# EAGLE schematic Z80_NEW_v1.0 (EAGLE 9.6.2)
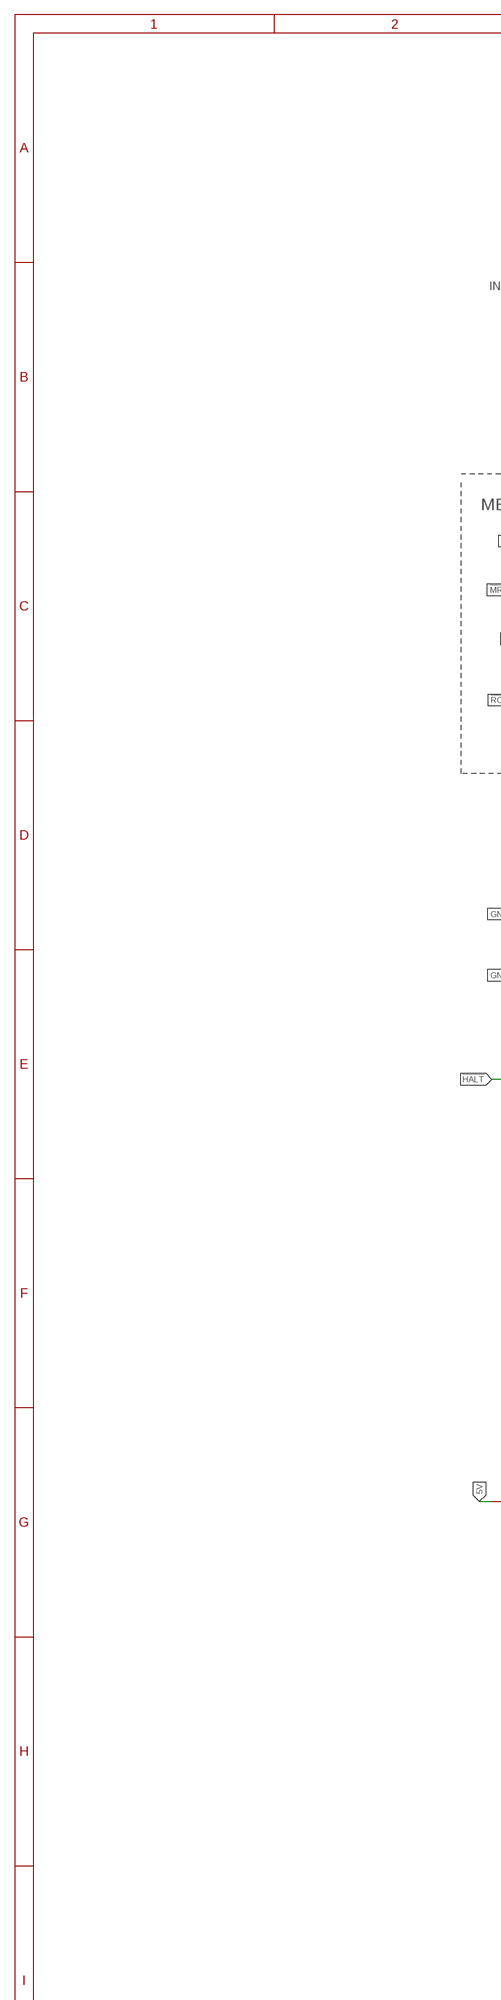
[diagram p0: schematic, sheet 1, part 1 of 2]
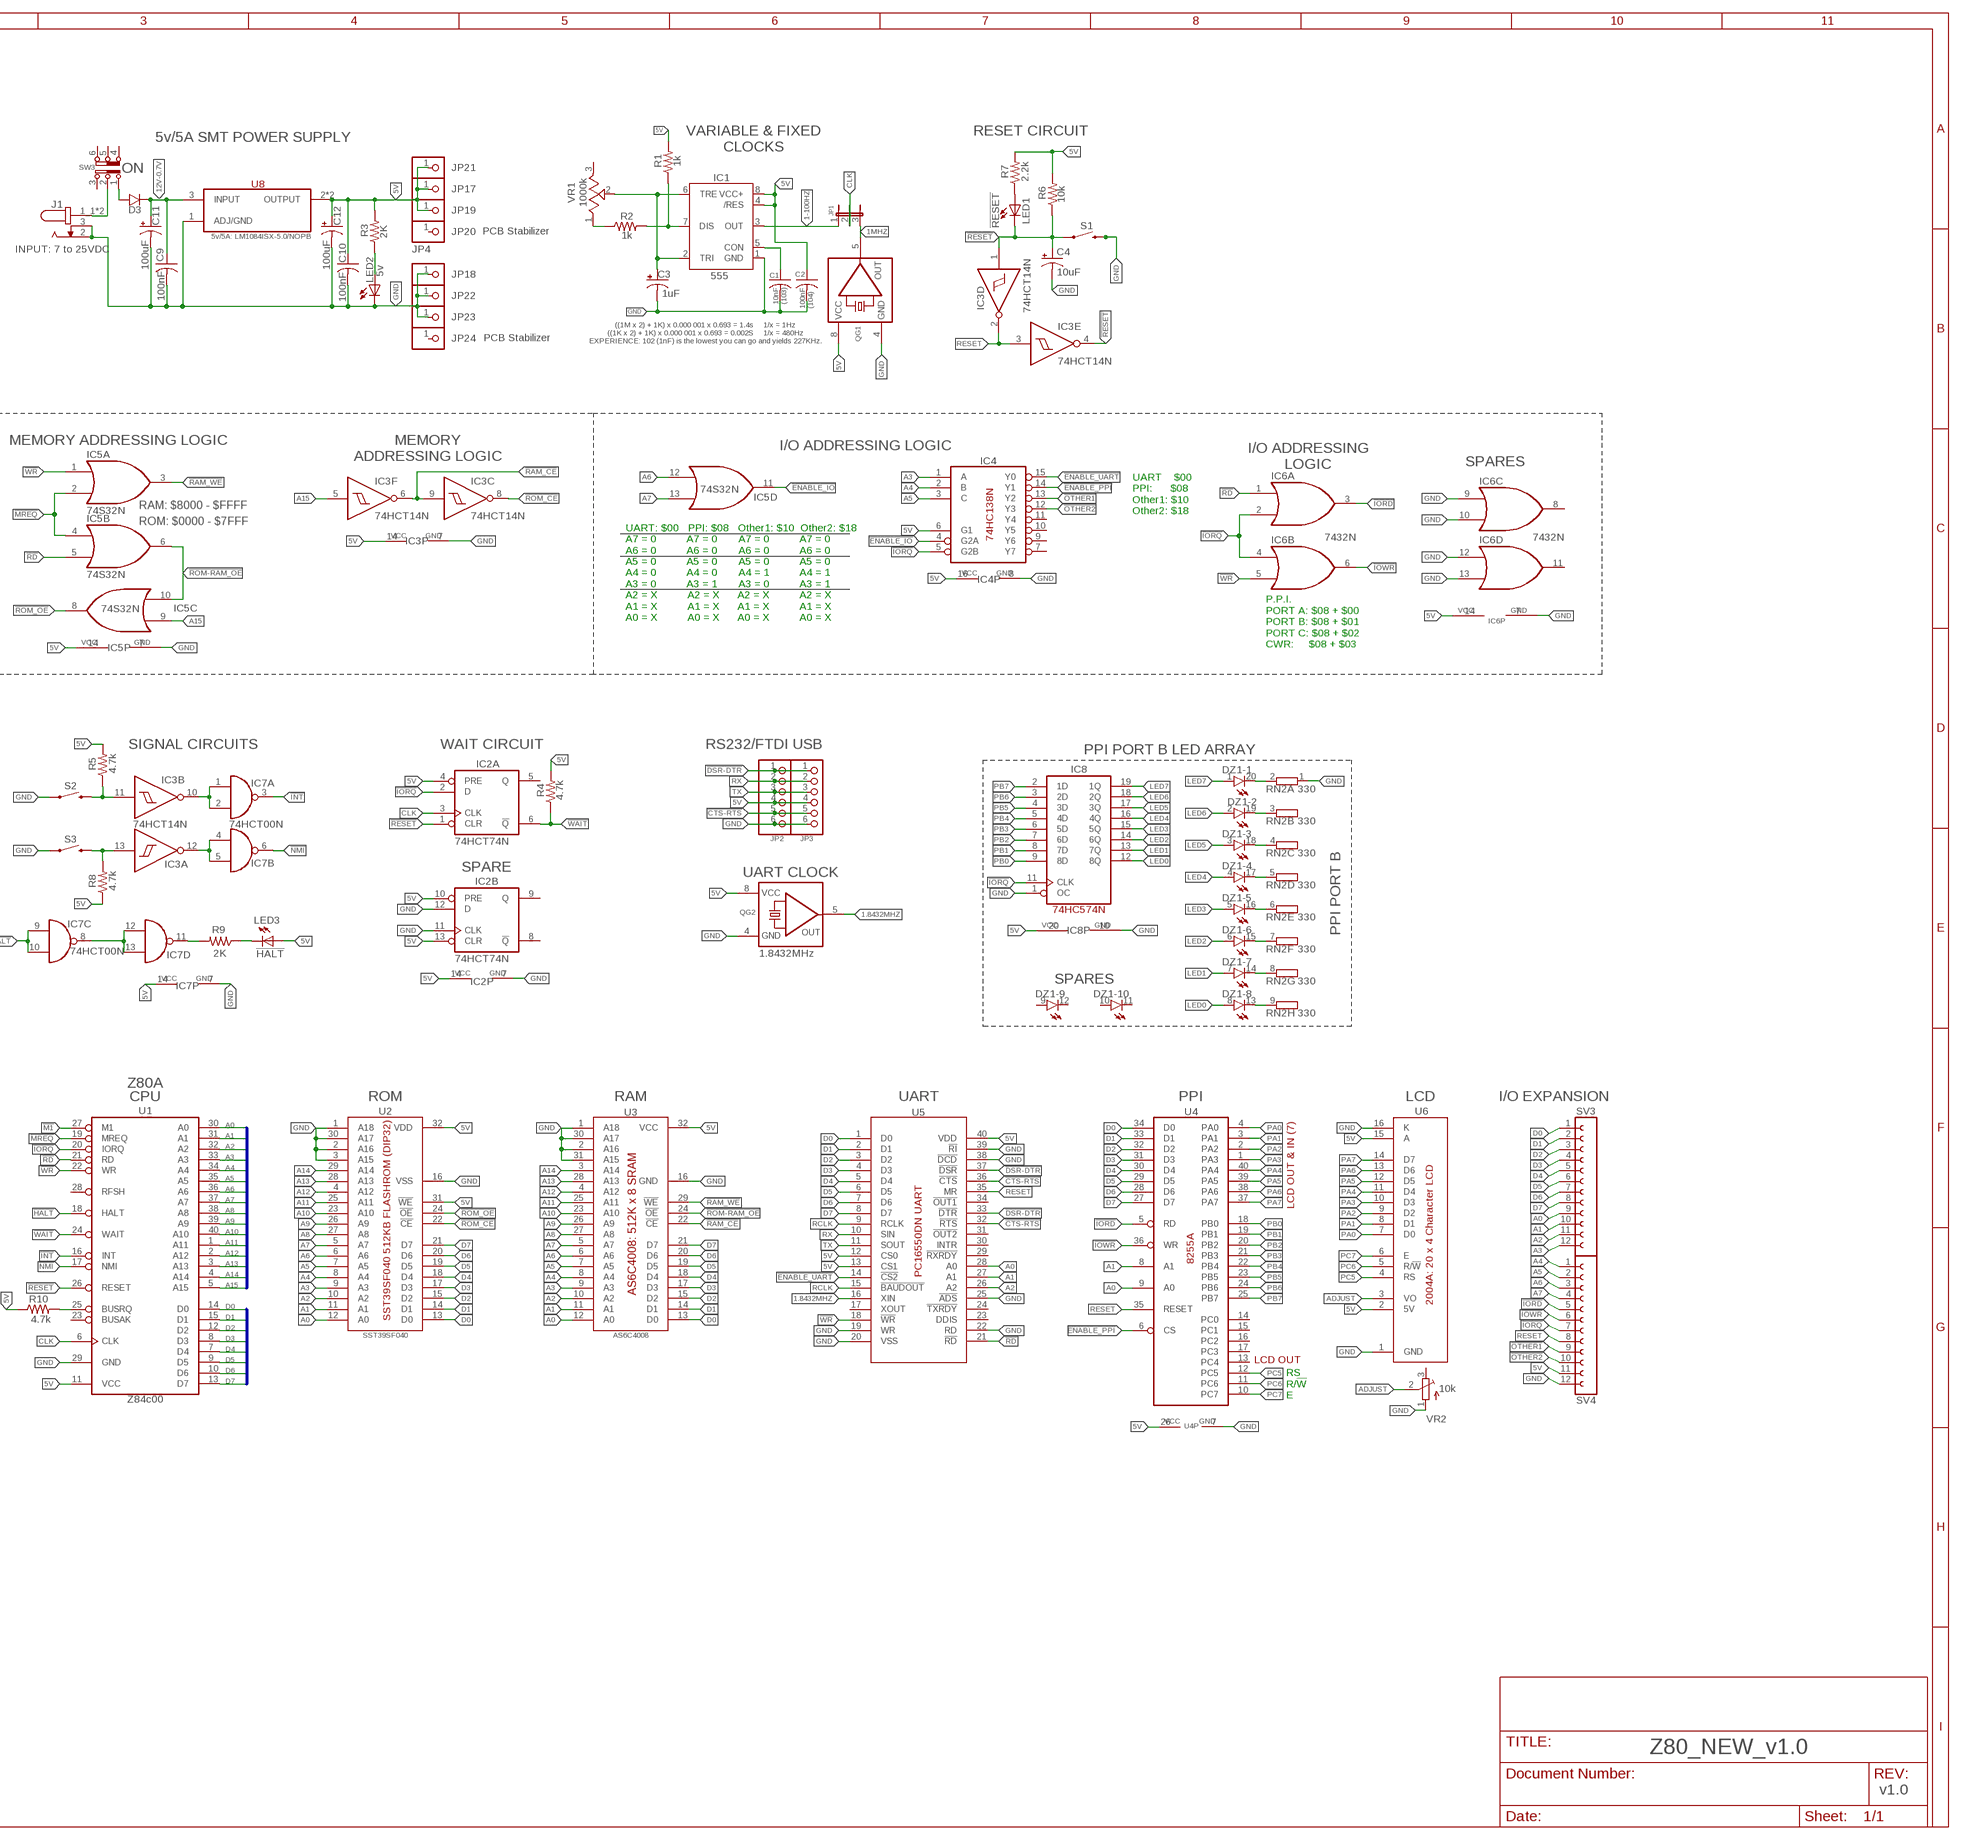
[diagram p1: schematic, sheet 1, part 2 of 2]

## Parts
C1  0.01uF  C-USC1206  [C1206]
C2  0.01uF  C-USC1206  [C1206]
C3  1uF  CPOL-USE2-5  [E2-5]
C4  10uF  CPOL-USE2-5  [E2-5]
C9  100nF  C-USC1206  [C1206]
C10  100nF  C-USC1206  [C1206]
C11  100uF  CPOL-USF  [PANASONIC_F]
C12  100uF  CPOL-USF  [PANASONIC_F]
D3  D1  DIODE_5V5A  [DIODE_5V5A]
DZ1  LB10  [LB10]
IC1  555  555P  [DIP08]
IC2  74HCT74N  [DIL14]
IC3  74HCT14N  [DIL14]
IC4  74HC138N  [DIL16]
IC5  74S32N  [DIL14]
IC6  7432N  [DIL14]
IC7  74HCT00N  [DIL14]
IC8  74HC574N  [DIL20]
J1  PRT-12748  [SPARKFUN_PRT-12748]
JP1  JP2E  [JP2]
JP2  PINHD-1X6  [1X06]
JP3  PINHD-1X6  [1X06]
JP17  PINHD-1X1  [1X01]
JP18  PINHD-1X1  [1X01]
JP19  PINHD-1X1  [1X01]
JP20  JP4  PINHD-1X1  [1X01]
JP21  PINHD-1X1  [1X01]
JP22  PINHD-1X1  [1X01]
JP23  PINHD-1X1  [1X01]
JP24  PINHD-1X1  [1X01]
LED1  !RESET!  LED3MM  [LED3MM]
LED2  5v  LEDCHIPLED_1206  [CHIPLED_1206]
LED3  !HALT!  LEDCHIPLED_1206  [CHIPLED_1206]
QG1  QG5460  [DIL08S]
QG2  1.8432MHz  QG5460  [DIL08S]
R1  1k  R-US_R1206  [R1206]
R2  1k  R-US_R1206  [R1206]
R3  2K  R-US_R1206  [R1206]
R4  4.7k  R-US_R1206  [R1206]
R5  4.7k  R-US_R1206  [R1206]
R6  10k  R-US_R1206  [R1206]
R7  2.2k  R-US_R1206  [R1206]
R8  4.7k  R-US_R1206  [R1206]
R9  2K  R-US_R1206  [R1206]
R10  4.7k  R-US_R1206  [R1206]
RN2  330  GE08R  [SIL9]
S1  MOMENTARY_SWITCH"  [MOMENTARY_SWITCH]
S2  MOMENTARY_SWITCH"  [MOMENTARY_SWITCH]
S3  MOMENTARY_SWITCH"  [MOMENTARY_SWITCH]
SV3  FE12W  [FE12W]
SV4  FE12W  [FE12W]
SW3  JS202011SCQN  [JS202011SCQN]
U1  Z80CPU  [DIL40]
U2  SST39SF040_DIP32  [DIL32]
U3  ALLIANCE_AS6C4008  [DIL32]
U4  8255A  [DIL40]
U5  PC16550DN/NOPB  [N40A]
U6  20X4LCD_2004A  [20X4LCD_2004A]
U8  LM1084ISX-5.0/NOPB  [TO254P1524X483-4N]
VR1  1000k  3352T-1-105LF  [TRIM_3352T-1-105LF]
VR2  10k  TRIMPOT3386  [TRIM-3386]

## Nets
1-100HZ: IC1.3(OUT) JP1.1
1.8432MHZ: QG2.5(OUT) U5.16(XIN)
1MHZ: JP1.3 QG1.5(OUT)
5V [Power]: C2.1 C10.1 C12.+ IC1.4(/RES) IC1.8(VCC+) IC2.4(A:PRE) IC2.10(B:PRE) IC2.13(B:CLR) IC2.14(P:VCC) IC3.14(P:VCC) IC4.6(G1) IC4.16(VCC) IC5.14(P:VCC) IC6.14(P:VCC) IC7.14(P:VCC) IC8.20(VCC) JP2.4 JP3.4 JP17.1 JP19.1 JP21.1 LED3.A QG1.8(VCC) QG2.8(VCC) R1.2 R3.2 R4.2 R5.2 R6.2 R7.2 R8.1 R10.1 SV4.11 U1.11(VCC) U2.31(!WE!) U2.32(VDD) U3.32(VCC) U4.26(VCC) U5.12(CS0) U5.13(CS1) U5.40(VDD) U6.2(5V) U6.15(A) U8.2(OUTPUT) U8.4(OUTPUT)
12V-0.7V: C9.1 C11.+ D3.C U8.3(INPUT)
!BUSRQ!: R10.2 U1.25(BUSRQ)
!CTS-RTS!: JP2.5 JP3.5 U5.32(!RTS) U5.36(!CTS)
!DSR-DTR!: JP2.1 JP3.1 U5.33(!DTR) U5.37(!DSR)
!ENABLE_IO!: IC4.4(G2A) IC5.11(D:O)
!ENABLE_PPI!: IC4.14(Y1) U4.6(CS)
!ENABLE_UART!: IC4.15(Y0) U5.14(!CS2)
!HALT!: IC7.9(C:I0) IC7.10(C:I1) U1.18(HALT)
!INT!: IC7.3(A:O) U1.16(INT)
!IORD!: IC6.3(A:O) SV4.5 U4.5(RD)
!IORQ!: IC2.2(A:D) IC4.5(G2B) IC6.2(A:I1) IC6.4(B:I0) IC8.11(CLK) SV4.7 U1.20(IORQ)
!IOWR!: IC6.6(B:O) SV4.6 U4.36(WR)
!M1!: U1.27(M1)
!MREQ!: IC5.2(A:I1) IC5.4(B:I0) U1.19(MREQ)
!NMI!: IC7.6(B:O) U1.17(NMI)
!OTHER1!: IC4.13(Y2) SV4.9
!OTHER2!: IC4.12(Y3) SV4.10
!RAM_CE!: IC3.6(F:O) IC3.9(C:I) U3.22(!CE!)
!RAM_WE!: IC5.3(A:O) U3.29(!WE!)
!RD!: IC5.5(B:I1) IC6.1(A:I0) U1.21(RD) U5.21(!RD)
!RESET!: C4.+ IC2.1(A:CLR) IC3.1(D:I) IC3.4(E:O) LED1.K(C) R6.1 S1.1 U1.26(RESET)
!ROM-RAM_OE!: IC5.6(B:O) IC5.10(C:I1) U3.24(!OE!)
!ROM_CE!: IC3.8(C:O) U2.22(!CE!)
!ROM_OE!: IC5.8(C:O) U2.24(!OE!)
!WAIT!: IC2.6(A:!Q) R4.1 U1.24(WAIT)
!WR!: IC5.1(A:I0) IC6.5(B:I1) U1.22(WR) U5.18(!WR)
A0: SV3.9 U1.30(A0) U2.12(A0) U3.12(A0) U4.9(A0) U5.28(A0)
A1: SV3.10 U1.31(A1) U2.11(A1) U3.11(A1) U4.8(A1) U5.27(A1)
A2: SV3.11 U1.32(A2) U2.10(A2) U3.10(A2) U5.26(A2)
A3: IC4.1(A) SV3.12 U1.33(A3) U2.9(A3) U3.9(A3)
A4: IC4.2(B) SV4.1 U1.34(A4) U2.8(A4) U3.8(A4)
A5: IC4.3(C) SV4.2 U1.35(A5) U2.7(A5) U3.7(A5)
A6: IC5.12(D:I0) SV4.3 U1.36(A6) U2.6(A6) U3.6(A6)
A7: IC5.13(D:I1) SV4.4 U1.37(A7) U2.5(A7) U3.5(A7)
A8: U1.38(A8) U2.27(A8) U3.27(A8)
A9: U1.39(A9) U2.26(A9) U3.26(A9)
A10: U1.40(A10) U2.23(A10) U3.23(A10)
A11: U1.1(A11) U2.25(A11) U3.25(A11)
A12: U1.2(A12) U2.4(A12) U3.4(A12)
A13: U1.3(A13) U2.28(A13) U3.28(A13)
A14: U1.4(A14) U2.29(A14) U3.3(A14)
A15: IC3.5(F:I) IC5.9(C:I0) U1.5(A15)
ADJUST: U6.3(VO) VR2.2(S)
CLK: IC2.3(A:CLK) JP1.2 U1.6(CLK)
D0: SV3.1 U1.14(D0) U2.13(D0) U3.13(D0) U4.34(D0) U5.1(D0)
D1: SV3.2 U1.15(D1) U2.14(D1) U3.14(D1) U4.33(D1) U5.2(D1)
D2: SV3.3 U1.12(D2) U2.15(D2) U3.15(D2) U4.32(D2) U5.3(D2)
D3: SV3.4 U1.8(D3) U2.17(D3) U3.17(D3) U4.31(D3) U5.4(D3)
D4: SV3.5 U1.7(D4) U2.18(D4) U3.18(D4) U4.30(D4) U5.5(D4)
D5: SV3.6 U1.9(D5) U2.19(D5) U3.19(D5) U4.29(D5) U5.6(D5)
D6: SV3.7 U1.10(D6) U2.20(D6) U3.20(D6) U4.28(D6) U5.7(D6)
D7: SV3.8 U1.13(D7) U2.21(D7) U3.21(D7) U4.27(D7) U5.8(D7)
GND [Power]: C1.2 C2.2 C3.- C4.- C9.2 C10.2 C11.- C12.- IC1.1(GND) IC2.7(P:GND) IC2.11(B:CLK) IC2.12(B:D) IC3.7(P:GND) IC4.8(GND) IC5.7(P:GND) IC6.7(P:GND) IC6.9(C:I0) IC6.10(C:I1) IC6.12(D:I0) IC6.13(D:I1) IC7.7(P:GND) IC8.1(OC) IC8.10(GND) J1.2 J1.3 JP2.6 JP3.6 JP18.1 JP22.1 JP23.1 LED2.C QG1.4(GND) QG2.4(GND) RN2.1 S1.3 S2.1 S3.1 SV4.12 U1.29(GND) U2.1(A18) U2.2(A16) U2.3(A15) U2.16(VSS) U2.30(A17) U3.1(A18) U3.2(A16) U3.16(GND) U3.30(A17) U3.31(A15) U4.7(GND) U5.19(WR) U5.20(VSS) U5.22(RD) U5.25(!ADS) U5.38(!DCD) U5.39(!RI) U6.1(GND) U6.16(K) U8.1(ADJ/GND) VR2.1(A)
LED0: DZ1.8(-8:A) IC8.12(8Q)
LED1: DZ1.7(-7:A) IC8.13(7Q)
LED2: DZ1.6(-6:A) IC8.14(6Q)
LED3: DZ1.5(-5:A) IC8.15(5Q)
LED4: DZ1.4(-4:A) IC8.16(4Q)
LED5: DZ1.3(-3:A) IC8.17(3Q)
LED6: DZ1.2(-2:A) IC8.18(2Q)
LED7: DZ1.1(-1:A) IC8.19(1Q)
N$1: LED1.A R7.1
N$2: IC1.7(DIS) R1.1 R2.2
N$3: C3.+ IC1.2(TRI) IC1.6(TRE) VR1.2(WIPER)
N$4: C1.1 IC1.5(CON)
N$5: D3.A SW3.1
N$6: R2.1 VR1.1(CCW)
N$8: J1.1_1 J1.1_2 SW3.2
N$9: LED2.A R3.1
N$10: IC3.10(B:O) IC7.1(A:I0) IC7.2(A:I1)
N$11: DZ1.20(-1:C) RN2.2
N$12: IC3.12(A:O) IC7.4(B:I0) IC7.5(B:I1)
N$13: DZ1.19(-2:C) RN2.3
N$14: IC7.8(C:O) IC7.12(D:I0) IC7.13(D:I1)
N$15: DZ1.18(-3:C) RN2.4
N$16: LED3.C R9.1
N$17: IC7.11(D:O) R9.2
N$18: DZ1.17(-4:C) RN2.5
N$19: IC3.11(B:I) R5.1 S2.3
N$20: IC3.13(A:I) R8.2 S3.3
N$22: DZ1.16(-5:C) RN2.6
N$23: DZ1.15(-6:C) RN2.7
N$24: DZ1.14(-7:C) RN2.8
N$25: DZ1.13(-8:C) RN2.9
PA0: U4.4(PA0) U6.7(D0)
PA1: U4.3(PA1) U6.8(D1)
PA2: U4.2(PA2) U6.9(D2)
PA3: U4.1(PA3) U6.10(D3)
PA4: U4.40(PA4) U6.11(D4)
PA5: U4.39(PA5) U6.12(D5)
PA6: U4.38(PA6) U6.13(D6)
PA7: U4.37(PA7) U6.14(D7)
PB0: IC8.9(8D) U4.18(PB0)
PB1: IC8.8(7D) U4.19(PB1)
PB2: IC8.7(6D) U4.20(PB2)
PB3: IC8.6(5D) U4.21(PB3)
PB4: IC8.5(4D) U4.22(PB4)
PB5: IC8.4(3D) U4.23(PB5)
PB6: IC8.3(2D) U4.24(PB6)
PB7: IC8.2(1D) U4.25(PB7)
PC5: U4.12(PC5) U6.4(RS)
PC6: U4.11(PC6) U6.5(R/!W!)
PC7: U4.10(PC7) U6.6(E)
RCLK: U5.9(RCLK) U5.15(!BAUDOUT)
RESET: IC3.2(D:O) IC3.3(E:I) SV4.8 U4.35(RESET) U5.35(MR)
RX: JP2.2 JP3.2 U5.10(SIN)
TX: JP2.3 JP3.3 U5.11(SOUT)
Unconnected: DZ1.9(-9:A) DZ1.10(-10:A) DZ1.11(-10:C) DZ1.12(-9:C) IC2.5(A:Q) IC2.8(B:!Q) IC2.9(B:Q) IC4.7(Y7) IC4.9(Y6) IC4.10(Y5) IC4.11(Y4) IC6.8(C:O) IC6.11(D:O) JP20.1 JP24.1 SW3.3 SW3.4 SW3.5 SW3.6 U1.23(BUSAK) U1.28(RFSH) U4.13(PC4) U4.14(PC0) U4.15(PC1) U4.16(PC2) U4.17(PC3) U5.17(XOUT) U5.23(DDIS) U5.24(!TXRDY) U5.29(!RXRDY) U5.30(INTR) U5.31(!OUT2) U5.34(!OUT1) VR1.3(CW) VR2.3(E)

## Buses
ADDRESSBUS:A0,A1,A2,A3,A4,A5,A6,A7,A8,A9,A10,A11,A12,A13,A14,A15
DATABUS:D0,D1,D2,D3,D4,D5,D6,D7

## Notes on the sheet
- RESET CIRCUIT
- 5v/5A SMT POWER SUPPLY
- VARIABLE & FIXED
  CLOCKS
- ON
- PCB Stabilizer
- 5v/5A: LM1084ISX-5.0/NOPB
- INPUT: 7 to 25VDC
- 10nF
  (103)
- 100nF
  (104)
- PCB Stabilizer
- ((1M x 2) + 1K) x 0.000 001 x 0.693 = 1.4s     1/x = 1Hz
  ((1K x 2) + 1K) x 0.000 001 x 0.693 = 0.002S     1/x = 480Hz
  EXPERIENCE: 102 (1nF) is the lowest you can go and yields 227KHz.
- MEMORY ADDRESSING LOGIC
- I/O ADDRESSING LOGIC
- I/O ADDRESSING
  LOGIC
- MEMORY
  ADDRESSING LOGIC
- SPARES
- RAM: $8000 - $FFFF
- UART    $00   
  PPI:      $08  
  Other1: $10  
  Other2: $18
- ROM: $0000 - $7FFF
- UART: $00   PPI: $08   Other1: $10  Other2: $18
  A7 = 0          A7 = 0       A7 = 0          A7 = 0 
  A6 = 0          A6 = 0       A6 = 0          A6 = 0
  A5 = 0          A5 = 0       A5 = 0          A5 = 0
  A4 = 0          A4 = 0       A4 = 1          A4 = 1
  A3 = 0          A3 = 1       A3 = 0          A3 = 1 
  A2 = X          A2 = X      A2 = X          A2 = X
  A1 = X          A1 = X      A1 = X          A1 = X
  A0 = X          A0 = X      A0 = X          A0 = X
- P.P.I.
  PORT A: $08 + $00
  PORT B: $08 + $01
  PORT C: $08 + $02
  CWR:     $08 + $03
- SIGNAL CIRCUITS | WAIT CIRCUIT | RS232/FTDI USB
- PPI PORT B LED ARRAY
- SPARE
- UART CLOCK
- PPI PORT B
- SPARES
- PPI | LCD
- Z80A
  CPU
- ROM | RAM | UART | I/O EXPANSION
- LCD OUT & IN (7)
- SST39SF040 | AS6C4008
- LCD OUT
- RS
  R/!W!
  E
- Z84c00
- v1.0

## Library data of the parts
C1 C2 C9 C10 = rcl:C-US: CAPACITOR, American symbol; SPICEPREFIX: C
C3 C4 C11 C12 = rcl:CPOL-US: POLARIZED CAPACITOR, American symbol; SPICEPREFIX: C
D3 = DIODE_5V5A:DIODE_5V5A: DIODE 5V/5A
DZ1 = led:LB10: LED BLOCK 10-LED bar graph, DIL, Siemens
IC1 = SparkFun-IC-Special-Function:555: General purpose bipolar Timer Datasheet SparkFun Products SparkFun SparkPunk Sequencer Kit (KIT-12707) Storefront Component: 555 Timer (COM-09273) Two parts valid for production: VFP: IC-11930 (M7555 PTH) VFP: IC-09173 (555 PTH) - Preferred; PROD_ID: IC-09173; PROD_ID_ALT: IC-09173
IC2 = 74xx-eu:74*74: Dual D type positive edge triggered FLIP FLOP, preset and clear
IC3 = 74xx-eu:74*14: Hex schmitt trigger INVERTER
IC4 = 74xx-eu:74*138: 3-line to 8-line DECODER/DEMULTIPLEXER
IC5 IC6 = 74xx-us:74*32: Quad 2-input OR gate
IC7 = 74xx-eu:74*00: Quad 2-input NAND gate
IC8 = 74xx-us:74*574: 8-bit D type FLIP FLOP bus driver
J1 = Jack_SMD_PRT-12748:PRT-12748: Check availability; AVAILABILITY: In Stock; DESCRIPTION: SparkFun Accessories DC Barrel Power Jack Connector SMD; MF: SparkFun; MP: PRT-12748; PACKAGE: None; PRICE: None; PURCHASE-URL: https://pricing.snapeda.com/search/part/PRT-12748/?ref=eda
JP1 = jumper:JP2E: JUMPER
JP2 JP3 = adafruit:PINHD-1X6: PIN HEADER
JP17-JP24 = adafruit:PINHD-1X1: Pin header 1x1 for 0.1" spacing
LED1-LED3 = adafruit:LED: LED
QG1 QG2 = crystal:QG5460: CRYSTAL RESONATOR; OC_FARNELL: unknown; OC_NEWARK: unknown
R1-R10 = rcl:R-US_: RESISTOR, American symbol; SPICEPREFIX: R
RN2 = resistor-sil:GE08R: SIL RESISTOR; OC_FARNELL: unknown; OC_NEWARK: unknown
S1-S3 = RBBB:MOMENTARY_SWITCH
SV3 SV4 = con-lsta:FE12W: FEMALE HEADER; OC_FARNELL: unknown; OC_NEWARK: unknown
SW3 = ck_switches:JS202011SCQN: DPDT SLIDE SWITCH
U1 = zilog:Z80CPU: Z80 FAMILY DEVICE
U2 = SST39SF040_DIP32:SST39SF040_DIP32: SST39SF040_DIP32
U3 = AS6C4008 512K x 8 SRAM DIL32:ALLIANCE_AS6C4008: Alliance Memory AS6C4008 512K x 8 SRAM DIL32
U4 = micro-intel:8255A: MICROCOMPUTER/PERIPHERAL DEVICE; OC_FARNELL: unknown; OC_NEWARK: unknown
U5 = TI_UART_pc16550D:PC16550DN/NOPB; MANUFACTURER_PART_NUMBER: PC16550DNNOPB; VENDOR: Texas Instruments
U6 = 20x4LCD_2004A:20X4LCD_2004A: 20 x 4 LCD Model 2004A
U8 = LM1084ISX-5.0_NOPB:LM1084ISX-5.0/NOPB: Check availability; AVAILABILITY: In Stock; DESCRIPTION: Linear Voltage Regulator IC Positive Fixed 1 Output 5A DDPAK/TO-263-3; MF: Texas Instruments; MP: LM1084ISX-5.0; PACKAGE: TO-263 Texas Instruments; PRICE: None; PURCHASE-URL: https://pricing.snapeda.com/search/part/LM1084ISX-5.0/?ref=eda
VR1 = Bourns_Trimpot_3352T-1-105LF:3352T-1-105LF: Check availability; AVAILABILITY: In Stock; DESCRIPTION: 1 MOhms 0.5W, 1/2W Through Hole Thumbwheel Potentiometer Top Adjustment; MF: Bourns; MP: 3352T-1-105LF; PACKAGE: 3352T-3 Bourns; PRICE: None; PURCHASE-URL: https://pricing.snapeda.com/search/part/3352T-1-105LF/?ref=eda
VR2 = adafruit:TRIMPOT: SMT trimmer potentiometer part number TC33X http://www.ladyada.net/library/eagle

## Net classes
0 default: clearance 0.254 mm
3 Power: width 0.254 mm, clearance 0.254 mm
